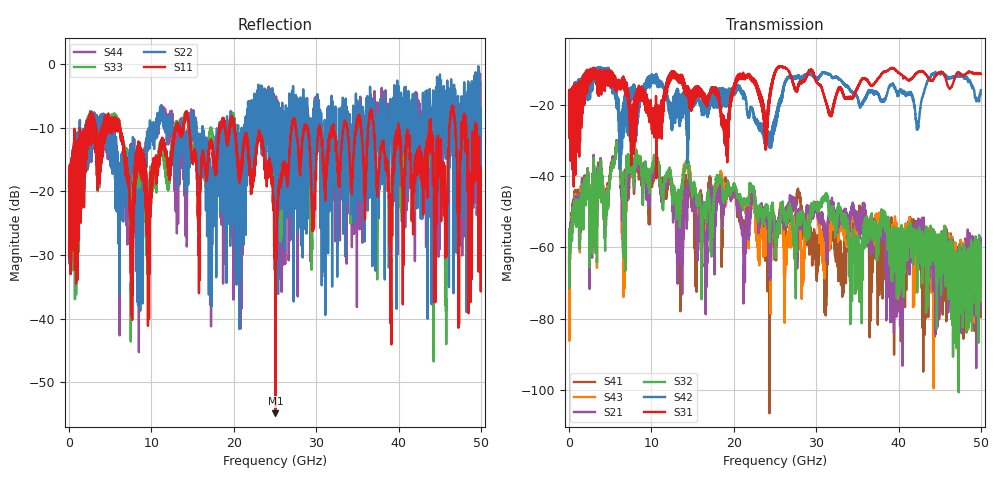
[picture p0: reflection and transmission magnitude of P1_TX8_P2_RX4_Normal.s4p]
!Keysight Technologies,N5225B,MY57041031,A.13.20.10
!Date: Friday, May 31, 2019 11:33:58
!Correction: S11(Full 4 Port(1,2,3,4))
!S12(Full 4 Port(1,2,3,4))
!S13(Full 4 Port(1,2,3,4))
!S14(Full 4 Port(1,2,3,4))
!S21(Full 4 Port(1,2,3,4))
!S22(Full 4 Port(1,2,3,4))
!S23(Full 4 Port(1,2,3,4))
!S24(Full 4 Port(1,2,3,4))
!S31(Full 4 Port(1,2,3,4))
!S32(Full 4 Port(1,2,3,4))
!S33(Full 4 Port(1,2,3,4))
!S34(Full 4 Port(1,2,3,4))
!S41(Full 4 Port(1,2,3,4))
!S42(Full 4 Port(1,2,3,4))
!S43(Full 4 Port(1,2,3,4))
!S44(Full 4 Port(1,2,3,4))
!S4P File: Measurements: <S11,S12,S13,S14>,
!<S21,S22,S23,S24>,
!<S31,S32,S33,S34>,
!<S41,S42,S43,S44>:
# Hz S  dB  R 50.0
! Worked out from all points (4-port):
!   5000 points, 10 MHz to 50 GHz, reference 50 ohm
!   strongest paths, dB at 10 MHz, 12.51 GHz, 25.01 GHz, 37.51 GHz, 50 GHz:
!     S31: -19.7, -10.8, -11.0, -12.7, -11.3
!     S42: -19.6, -27.2, -24.0, -17.1, -15.9
!     S32: -54.9, -43.1, -57.6, -56.1, -60.5
!     S21: -63.8, -42.7, -54.4, -56.6, -69.5
!     S43: -61.1, -44.1, -53.4, -55.2, -65.3
!     S41: -62.8, -41.5, -59.0, -69.9, -66.1
!   lowest |S11| = -54.9 dB at 25.05 GHz (marker M1), VSWR 1.00, Z = 49.8 + j0.0417 ohm
!   |S11| at or under -10 dB: 6.192 GHz to 12.89 GHz (6.696 GHz wide, 70.2 % of centre); 20.1 GHz to 26.99 GHz (6.892 GHz wide, 29.3 % of centre); 40 GHz to 43.77 GHz (3.765 GHz wide, 8.99 % of centre)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
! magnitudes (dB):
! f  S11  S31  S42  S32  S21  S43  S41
! 10 MHz  -19.4  -19.7  -19.6  -54.9  -63.8  -61.1  -62.8
! 5.92 GHz  -10.2  -14.9  -19.6  -31.1  -30.8  -31.4  -31.1
! 6.68 GHz  -13.1  -12.6  -24.1  -50.7  -49.7  -55.0  -45.3
! 25.05 GHz  -54.9  -10.5  -25.0  -59.4  -54.1  -52.8  -57.0
! 27.29 GHz  -8.6  -14.5  -12.2  -57.8  -47.6  -53.1  -48.8
! 31.12 GHz  -20.7  -18.6  -10.9  -45.1  -58.2  -58.3  -65.5
! 50 GHz  -22.6  -11.3  -15.9  -60.5  -69.5  -65.3  -66.1
